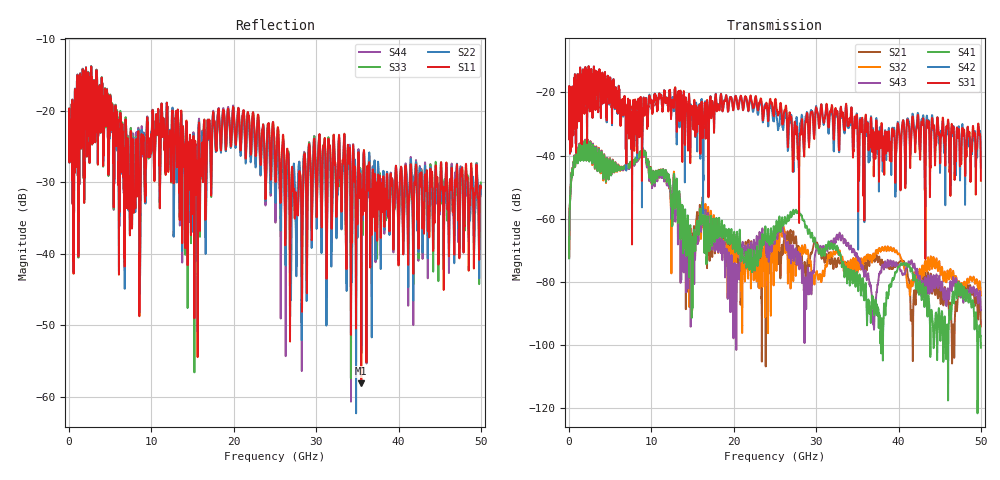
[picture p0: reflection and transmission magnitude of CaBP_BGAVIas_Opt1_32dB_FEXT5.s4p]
!* Samtec Inc. NovaRay Examax Flyover System  *
!*  REV DATE  = 08/08/18  *
!*  TYPE  = TOUCHSTONE  *
!*  PORTS  = 4 port  *
!*  UNITS  = GHz  *
!*  DATA RANGE = DC  to 50 GHz; 10 MHz Step  *
!*  PARAMETER  = S  *
!*  FORMAT  = Real-Imaginary  *
!*  REFERENCE  = 50 ohms  *
!*  SOURCE  = HFSS  *
!*  VALIDATED  = No  *
!*  MANUFACTURER = SAMTEC  *
!*  INTERCONNECT = NVAx to EBCx to EBCx to NVAx  *
!*  [Full Channel NVAx to EBCx to EBCx to NVAx  with PCB Trace and BGA Via]  *
!*  BOUNDARY A  = Silicon BGA Ball Pad  *
!*  BOUNDARY B  = Silicon BGA Ball Pad  *
!*  NVAx (end a) ->>- (end b) NVAx  *
!*  Port 01 ->>- Port 02  *
!*  Port 03 ->>- Port 04  *
!***************************** CHANNEL MODEL ******************************************
# GHz S RI R 50
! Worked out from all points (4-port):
!   5000 points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, 10 MHz to 50 GHz, reference 50 ohm
!   strongest paths, dB at 10 MHz, 12.51 GHz, 25.01 GHz, 37.51 GHz, 50 GHz:
!     S31: -23.1, -22.6, -22.3, -32.5, -48.0
!     S42: -23.1, -22.6, -23.8, -34.8, -43.7
!     S41: -72.7, -60.3, -66.3, -89.9, -101.0
!     S43: -72.4, -57.1, -66.7, -80.5, -89.1
!     S32: -72.3, -59.5, -66.5, -71.0, -84.4
!     S21: -72.5, -60.0, -72.1, -73.7, -94.2
!   lowest |S11| = -58.1 dB at 35.48 GHz (marker M1), VSWR 1.00, Z = 50.1 + j0.0131 ohm
!   |S11| at or under -10 dB: start of sweep to end of sweep
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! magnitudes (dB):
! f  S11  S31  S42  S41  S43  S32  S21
! 10 MHz  -21.4  -23.1  -23.1  -72.7  -72.4  -72.3  -72.5
! 1.1 GHz  -17.8  -15.8  -15.8  -41.1  -40.9  -40.9  -41.0
! 9.03 GHz  -24.1  -23.5  -23.7  -39.0  -39.5  -39.4  -38.9
! 14.4 GHz  -40.4  -31.4  -31.5  -59.3  -64.0  -70.8  -77.5
! 27.7 GHz  -33.3  -35.0  -30.2  -58.3  -70.7  -71.7  -70.5
! 35.48 GHz  -58.1  -32.6  -32.5  -82.2  -75.0  -72.9  -74.9
! 50 GHz  -30.6  -48.0  -43.7  -101.0  -89.1  -84.4  -94.2
